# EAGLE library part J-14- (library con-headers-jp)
HEADER JACK PINS
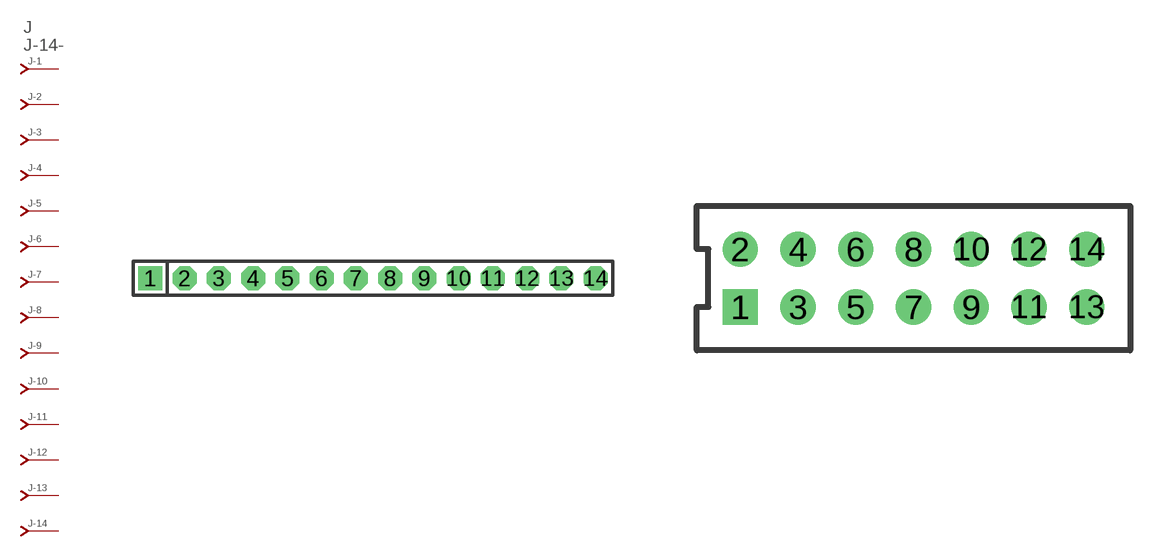
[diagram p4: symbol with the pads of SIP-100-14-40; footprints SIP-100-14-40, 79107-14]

Designator prefix J; gates -2=J-N -3=J-N -4=J-N -5=J-N -6=J-N -7=J-N -8=J-N -9=J-N -10=J-N -11=J-N -12=J-N -13=J-N -14=J-N -1=J-NV

## J-14-SIP-100-40  [SIP-100-14-40]
1  -1:J  pas
2  -2:J  pas
3  -3:J  pas
4  -4:J  pas
5  -5:J  pas
6  -6:J  pas
7  -7:J  pas
8  -8:J  pas
9  -9:J  pas
10  -10:J  pas
11  -11:J  pas
12  -12:J  pas
13  -13:J  pas
14  -14:J  pas

## J-14-79107  [79107-14]
Pads as for SIP-100-14-40

## J-14-79109  [79109-14]
Pads as for SIP-100-14-40

## J-14-87264  [87264-14]
Pads as for SIP-100-14-40

## J-14-87340  [87340-14]
Pads as for SIP-100-14-40

## J-14-87368  [87368-14]
Pads as for SIP-100-14-40

## J-14-535512  [535512-14]
Pads as for SIP-100-14-40

## J-14-100-2X07  [DIL-100-2X07]
Pads as for SIP-100-14-40

## J-14-100-2X07_M  [DIL-100-2X07_M]
Pads as for SIP-100-14-40

## J-14-2MM-2X07  [DIL-2MM-2X07]
Pads as for SIP-100-14-40

## J-14-2MM-2X07_M  [DIL-2MM-2X07_M]
Pads as for SIP-100-14-40

## J-14-SIP-100-32  [SIP-100-14-32]
Pads as for SIP-100-14-40

## J-14-SIP-100-40Y  [SIP-100-14-40Y]
Pads as for SIP-100-14-40

## J-14-SIP-100-32Y  [SIP-100-14-32Y]
Pads as for SIP-100-14-40

## J-14-71991  [71991-14]
Pads as for SIP-100-14-40

## J-14-KK-4455-B14  [KK-4455-B14]
Pads as for SIP-100-14-40

## J-14-KK-4455-A14  [KK-4455-A14]
Pads as for SIP-100-14-40

## J-14-KK-4455-C14  [KK-4455-C14]
Pads as for SIP-100-14-40

## Footprint SIP-100-14-40 (pad centres in mm)
SIP Header - 0.1", 40 mil drill
drill 1.016 pad 1.778 square: 1 -16.51,0
drill 1.016 pad 1.778 octagon: 2 -13.97,0; 3 -11.43,0; 4 -8.89,0; 5 -6.35,0; 6 -3.81,0; 7 -1.27,0; 8 1.27,0; 9 3.81,0; 10 6.35,0; 11 8.89,0; 12 11.43,0; 13 13.97,0; 14 16.51,0

## Footprint 79107-14 (pad centres in mm)
Molex Board-To-Board Receptacal 2.00mm (.079") Pitch Milli-Grid Header, Vertical, Through-Hole Mates with: 87759, 87762, 87758, 87760
drill 0.711 square: 1 -6,-1
drill 0.711: 2 -6,1; 3 -4,-1; 4 -4,1; 5 -2,-1; 6 -2,1; 7 0,-1; 8 0,1; 9 2,-1; 10 2,1; 11 4,-1; 12 4,1; 13 6,-1; 14 6,1

## Footprint 79109-14 (pad centres in mm)
Molex Board-to-Board Receptacal 2.00mm (.079") Pitch Milli-Grid Header, Vertical, Top/Bottom Entry Mates with: 87758, 87759, 87760, 87831, 87832, 87833
smd 1.12 x 1.83: 1 -6,-2.65; 2 -6,2.65; 3 -4,-2.65; 4 -4,2.65; 5 -2,-2.65; 6 -2,2.65; 7 0,-2.65; 8 0,2.65; 9 2,-2.65; 10 2,2.65; 11 4,-2.65; 12 4,2.65; 13 6,-2.65; 14 6,2.65
hole 0.914 at -5,0
hole 0.914 at -6,1
hole 0.914 at -6,-1
hole 0.914 at -4,-1
hole 0.914 at -4,1
hole 0.914 at -2,-1
hole 0.914 at -2,1
hole 0.914 at 5,0
hole 0.914 at 0,1
hole 0.914 at 0,-1
hole 0.914 at 2,1
hole 0.914 at 2,-1
hole 0.914 at 4,1
hole 0.914 at 4,-1
hole 0.914 at 6,1
hole 0.914 at 6,-1

## Footprint 87264-14 (pad centres in mm)
Molex Board-To-Board Receptacal 2.00mm (.079") Pitch Milli-Grid Header, Side Entry Mates with 2mm(.079") Mill-Grid Header
drill 0.914 square: 1 -6,-2.25
drill 0.914: 2 -6,2.25; 3 -4,-2.25; 4 -4,2.25; 5 -2,-2.25; 6 -2,2.25; 7 0,-2.25; 8 0,2.25; 9 2,-2.25; 10 2,2.25; 11 4,-2.25; 12 4,2.25; 13 6,-2.25; 14 6,2.25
